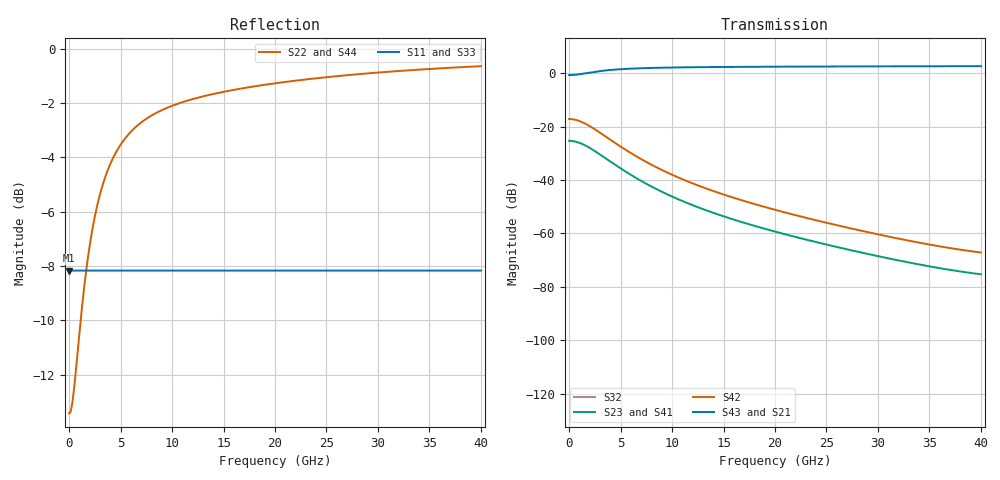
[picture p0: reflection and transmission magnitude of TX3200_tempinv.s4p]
# hz S ri R 50
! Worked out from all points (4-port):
!   20000 points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, 2 MHz to 40 GHz, reference 50 ohm
!   strongest paths, dB at 2 MHz, 10 GHz, 20 GHz, 30 GHz, 40 GHz:
!     S43: -0.7, 2.2, 2.5, 2.6, 2.7
!     S21: -0.8, 2.1, 2.4, 2.6, 2.7
!     S42: -17.1, -38.0, -51.1, -60.3, -67.1
!     S23: -25.3, -46.2, -59.3, -68.5, -75.3
!     S41: -25.3, -46.2, -59.3, -68.5, -75.3
!     S32: -, -, -, -, -
!   lowest |S11| = -8.2 dB at 2 MHz (marker M1), VSWR 2.28, Z = 114 + j0 ohm
!   |S11| at or under -10 dB: nowhere
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2000000  0.3907 0  0 0  0 0  0 0
         0.9166 0.00024  0.2134 -0.000614  -0.0544 7.02e-05  0.1392 -0.00018
         0 0  0 0  0.3907 0  0 0
         -0.0544 7.02e-05  0.1392 -0.00018  0.9231 0.000232  0.1968 -0.000594
1.478e9  0.3907 0  0 0  0 0  0 0
         0.9774 0.1412  0.0578 -0.3614  -0.0293 0.0347  0.075 -0.0889
         0 0  0 0  0.3907 0  0 0
         -0.0293 0.0347  0.075 -0.0889  0.9809 0.138  0.049 -0.3532
2.87e9  0.3907 0  0 0  0 0  0 0
        1.072 0.1933  -0.1841 -0.4947  -0.0023 0.0313  0.00588 -0.08
        0 0  0 0  0.3907 0  0 0
        -0.0023 0.0313  0.00588 -0.08  1.073 0.1917  -0.1861 -0.4907
5.624e9  0.3907 0  0 0  0 0  0 0
         1.193 0.1888  -0.4938 -0.4832  0.00863 0.0109  -0.0221 -0.0278
         0 0  0 0  0.3907 0  0 0
         0.00863 0.0109  -0.0221 -0.0278  1.195 0.1902  -0.4988 -0.4868
9.502e9  0.3907 0  0 0  0 0  0 0
         1.262 0.1537  -0.6718 -0.3935  0.00501 0.00213  -0.0128 -0.00545
         0 0  0 0  0.3907 0  0 0
         0.00501 0.00213  -0.0128 -0.00546  1.267 0.1543  -0.6831 -0.3948
2.1996e10  0.3907 0  0 0  0 0  0 0
           1.326 0.1014  -0.8343 -0.2596  0.000831 -0.00022  -0.00213 0.000564
           0 0  0 0  0.3907 0  0 0
           0.000832 -0.000219  -0.00213 0.000561  1.329 0.0981  -0.8409 -0.251
4e10  0.3907 0  0 0  0 0  0 0
      1.356 0.0726  -0.9104 -0.1857  4.33e-05 -0.000167  -0.000111 0.000427
      0 0  0 0  0.3907 0  0 0
      4.38e-05 -0.000167  -0.000112 0.000426  1.355 0.0703  -0.9098 -0.1799
